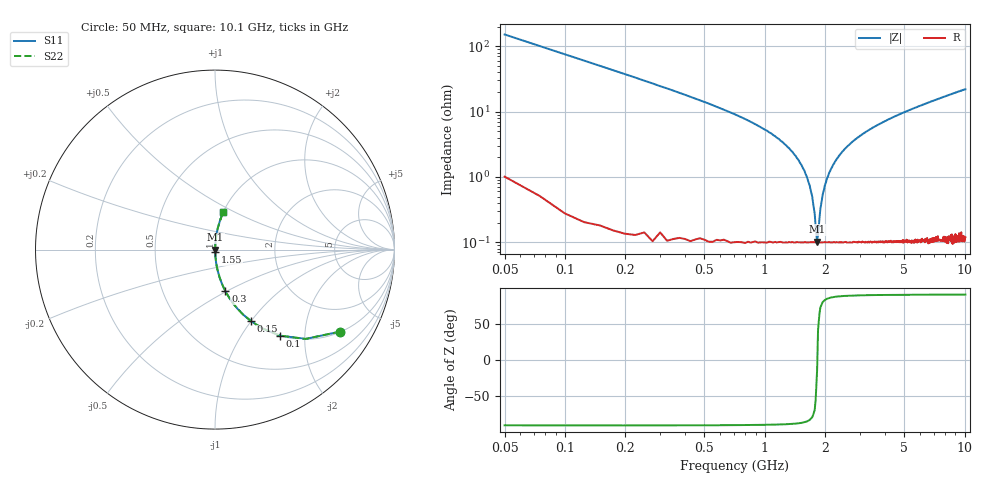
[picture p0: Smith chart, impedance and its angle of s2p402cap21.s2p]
! AVX Thin Film Operation		Date: April 2003
! Description: Accu-P® Series, Thin Film, SMD, RF Capacitor
! Part Number: 0402ZK210FBW
! 50 MHz  -  10.05 GHz
! Serial Measurements
# hz S db R 50
!	S11		S21		S12		S22
!	dB	Phase	dB	Phase	dB	Phase	dB	Phase
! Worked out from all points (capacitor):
!   400 points, 50 MHz to 10.1 GHz, reference 50 ohm
!   read as one part in series: C = 21 pF near 100 MHz
!   lowest |Z| = 103 mohm at 1.83 GHz (marker M1)
!   series resonance near 1.834 GHz, so ESL is about 360 pH
!   S11 on the Smith chart (normalised r, x): 50 MHz: 1.02, -3.03; 100 MHz: 1.01, -1.51; 150 MHz: 1.00, -1.00; 300 MHz: 1.00, -0.49; 1.55 GHz: 1.00, -0.03; 10.1 GHz: 1.00, +0.44
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5e7  -1.59 -33.3  -5.20 56.3  -5.20 56.3  -1.59 -33.3
1e8  -4.41 -52.8  -1.98 37.0  -1.98 37.0  -4.41 -52.8
1.5e8  -6.98 -63.2  -0.99 26.6  -0.99 26.6  -6.98 -63.2
3e8  -12.50 -75.9  -0.27 13.8  -0.27 13.8  -12.50 -75.9
6.25e8  -19.50 -83.3  -0.06 6.1  -0.06 6.1  -19.50 -83.3
1.23e9  -29.30 -86.4  -0.01 1.9  -0.01 1.9  -29.30 -86.4
1.55e9  -37.20 -85.1  -0.01 0.8  -0.01 0.8  -37.20 -85.1
1.63e9  -40.10 -83.7  -0.01 0.6  -0.01 0.6  -40.10 -83.7
1.73e9  -46.00 -78.2  -0.01 0.3  -0.01 0.3  -46.00 -78.2
1.78e9  -51.30 -68.4  -0.01 0.1  -0.01 0.1  -51.30 -68.4
1.83e9  -59.80 -13.9  -0.01 0.0  -0.01 0.0  -59.80 -13.9
1.9e9  -49.80 71.9  -0.01 -0.2  -0.01 -0.2  -49.80 71.9
1.95e9  -45.50 78.9  -0.01 -0.3  -0.01 -0.3  -45.50 78.9
2.05e9  -40.50 83.4  -0.01 -0.5  -0.01 -0.5  -40.50 83.4
2.2e9  -36.30 85.4  -0.01 -0.9  -0.01 -0.9  -36.30 85.4
2.45e9  -32.20 86.3  -0.01 -1.4  -0.01 -1.4  -32.20 86.3
2.7e9  -29.60 86.4  -0.01 -1.9  -0.01 -1.9  -29.60 86.4
3.4e9  -25.30 85.8  -0.02 -3.1  -0.02 -3.1  -25.30 85.8
5.08e9  -20.10 83.7  -0.05 -5.7  -0.05 -5.7  -20.10 83.7
6.75e9  -17.10 81.5  -0.10 -8.0  -0.10 -8.0  -17.10 81.5
8.43e9  -15.00 79.4  -0.15 -10.3  -0.15 -10.3  -15.00 79.4
1.01e10  -13.40 77.3  -0.21 -12.4  -0.21 -12.4  -13.40 77.3
